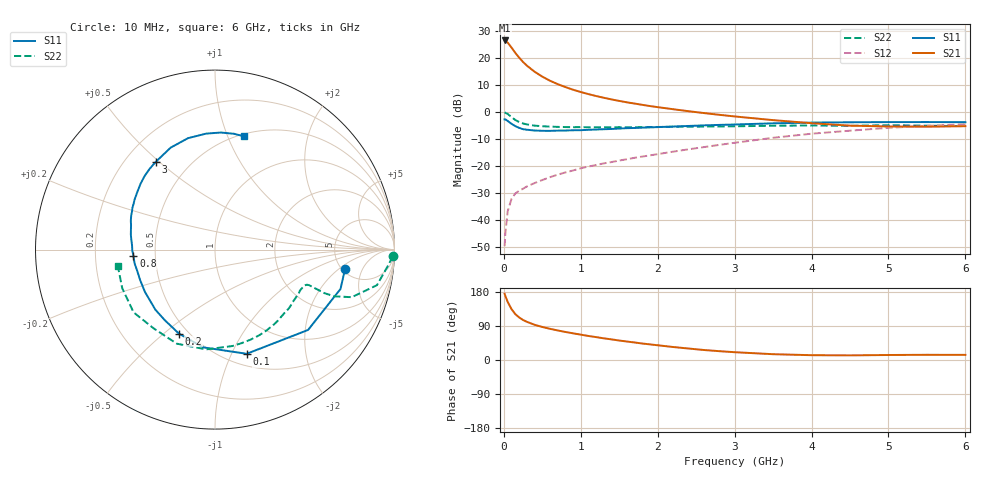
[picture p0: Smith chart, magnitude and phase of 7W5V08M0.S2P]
! Infineon Technologies  Discrete & RF Semiconductors
! BFS17W
! Si NPN RF Bipolar Junction Transistor in SOT323
! VCE = 5 V  IC = 8 mA
! Common Emitter S-Parameters:  August  1999
# GHz  S  MA  R  50
!  f  S11  S21  S12  S22
! GHz  MAG  ANG  MAG  ANG  MAG  ANG  MAG  ANG
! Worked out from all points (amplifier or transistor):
!   36 points, 10 MHz to 6 GHz, reference 50 ohm
!   highest |S21| = 26.5 dB at 10 MHz (marker M1)
!   |S21| within 3 dB of that: start of sweep to 108.8 MHz
!   unconditionally stable (mu >= 1): 459.3 MHz to 2.376 GHz; 5.104 GHz to end of sweep
!   at 250 MHz: K = 0.73, MSG = 23.5 dB, |S12| = -28.4 dB
!   at 1.4 GHz: K = 1.20, MAG = 8.9 dB, |S12| = -18.5 dB
!   at 6 GHz: K = 1.06, MAG = -1.8 dB, |S12| = -4.5 dB
!   S11 on the Smith chart (normalised r, x): 10 MHz: 5.31, -2.45; 100 MHz: 0.62, -1.14; 200 MHz: 0.45, -0.56; 800 MHz: 0.37, -0.03; 3 GHz: 0.32, +0.49; 6 GHz: 0.53, +1.15
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0.01  0.7326 -8.4  21.17 174.7  0.0033 78.8  0.9912 -2.2
0.02  0.7329 -17.4  20.91 168.8  0.0058 87.3  0.9675 -5.4
0.05  0.6851 -40.8  19.32 153.3  0.0146 73.2  0.9237 -12.4
0.1  0.6067 -73.1  15.61 134.1  0.0248 59.9  0.8065 -19.2
0.15  0.5486 -96.9  12.43 120.8  0.0313 54.1  0.7131 -21.4
0.2  0.5095 -113.2  10.15 112.1  0.035 53.8  0.6545 -21.7
0.25  0.4825 -125.5  8.463 105.6  0.0382 52.4  0.6149 -21.3
0.3  0.4718 -134.7  7.233 100.7  0.0421 53.3  0.592 -21.1
0.4  0.4561 -148.7  5.583 92.9  0.0486 55.9  0.5612 -20.7
0.5  0.4504 -157.8  4.531 87.2  0.0553 57.8  0.5478 -20.9
0.6  0.4493 -164.7  3.803 82.3  0.0624 60.0  0.5383 -21.7
0.8  0.4556 -175.4  2.905 74.0  0.0764 63.0  0.5285 -24.5
0.9  0.461 -179.5  2.594 70.4  0.0831 63.9  0.5253 -26.0
1.1  0.4702 172.9  2.151 63.4  0.0982 65.5  0.5242 -29.9
1.3  0.4821 166.3  1.841 57.2  0.1124 66.5  0.5223 -34.4
1.6  0.5037 158.0  1.515 48.7  0.1342 67.8  0.5235 -41.3
2.2  0.5396 143.2  1.131 34.3  0.1852 69.6  0.534 -57.1
3  0.5896 124.2  0.831 20.6  0.2706 67.7  0.5459 -79.8
3.5  0.6195 113.5  0.71 15.3  0.3345 64.0  0.5584 -95.2
4.5  0.648 94.4  0.561 12.2  0.4528 52.0  0.5563 -127.8
5.5  0.6539 80.7  0.536 13.7  0.5565 39.0  0.5598 -157.4
6  0.6513 75.4  0.549 13.5  0.5971 32.7  0.5491 -170.5
